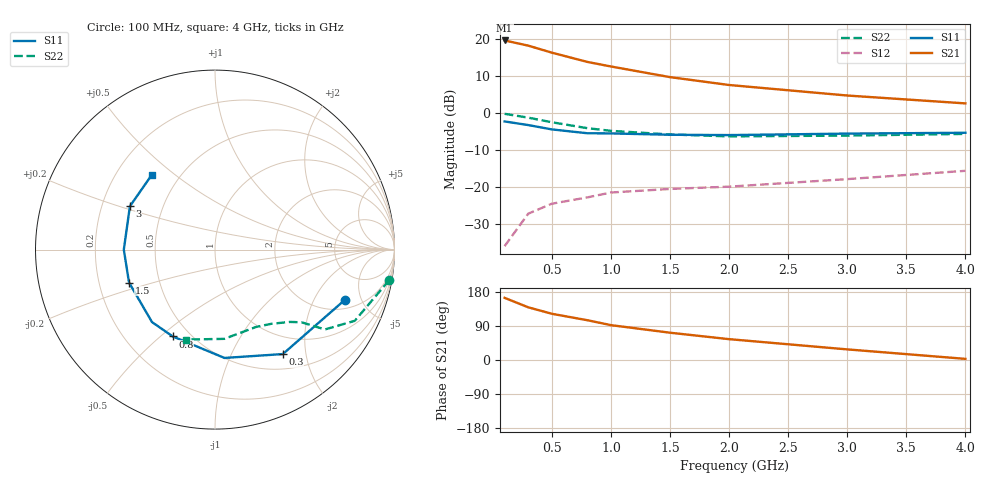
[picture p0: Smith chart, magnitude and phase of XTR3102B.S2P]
! HXTR-3102 Common Emitter
! Vce=15V  Ic=30mA
# ghz s ma r 50
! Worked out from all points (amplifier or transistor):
!   9 points, 100 MHz to 4 GHz, reference 50 ohm
!   highest |S21| = 19.7 dB at 100 MHz (marker M1)
!   |S21| within 3 dB of that: start of sweep to 468.4 MHz
!   unconditionally stable (mu >= 1): 1.847 GHz to 3.466 GHz
!   at 300 MHz: K = 0.23, MSG = 22.7 dB, |S12| = -27.1 dB
!   at 1 GHz: K = 0.67, MSG = 17.0 dB, |S12| = -21.4 dB
!   at 4 GHz: K = 0.94, MSG = 9.1 dB, |S12| = -15.5 dB
!   S11 on the Smith chart (normalised r, x): 100 MHz: 2.59, -3.64; 300 MHz: 0.71, -1.60; 800 MHz: 0.40, -0.55; 1.5 GHz: 0.33, -0.17; 3 GHz: 0.32, +0.22; 4 GHz: 0.35, +0.42
0.1  0.777 -21.0  9.661 164.0  0.016 71.0  0.985 -10.0
0.3  0.694 -57.0  8.222 139.0  0.044 58.0  0.874 -27.0
0.5  0.606 -85.0  6.607 122.0  0.06 48.0  0.757 -36.0
0.8  0.538 -116.0  4.955 105.0  0.073 40.0  0.63 -40.0
1  0.535 -131.0  4.296 92.0  0.085 34.0  0.58 -44.0
1.5  0.513 -159.0  3.086 72.0  0.095 32.0  0.518 -53.0
2  0.508 -180.0  2.415 55.0  0.102 31.0  0.488 -62.0
3  0.532 153.0  1.74 28.0  0.129 33.0  0.5 -84.0
4  0.546 130.0  1.362 3.0  0.167 29.0  0.527 -108.0
